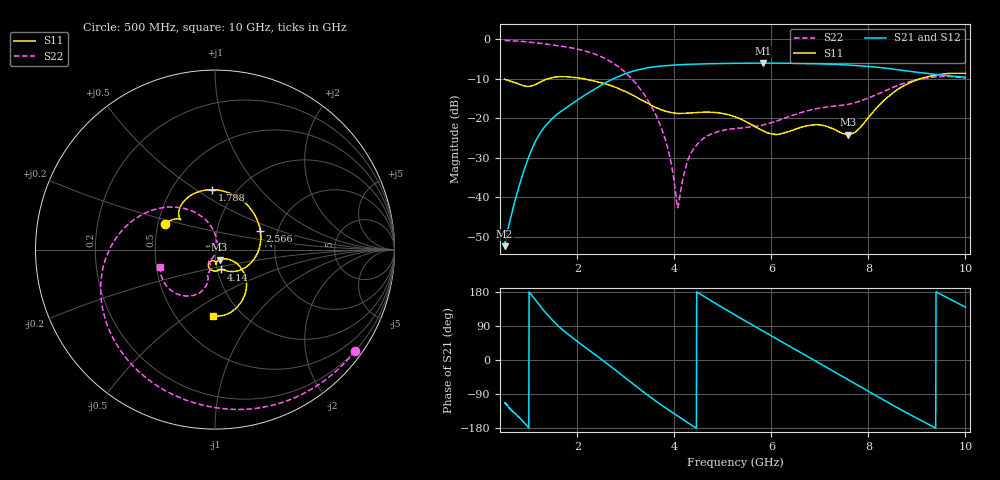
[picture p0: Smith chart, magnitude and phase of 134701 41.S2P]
!  2-Port S-parameters saved by WinCal
! VAR MeasName=S-Parameters (CALIBRATED_DATA) read from VNA (N5242A)
! VAR MeasDate=2013-7-3 16:37:49
! VAR NAME=134701 41
! VAR FILENAME=134701 41.S2P
! VAR DATE=2013-7-3 16:37:49
! VAR PHYS_PORTS=1,2
# Hz S MA R 50
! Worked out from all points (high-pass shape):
!   1601 points, 500 MHz to 10 GHz, reference 50 ohm
!   highest |S21| = -6.05 dB at 5.832 GHz (marker M1); lowest = -52.3 dB at 500 MHz (marker M2)
!   |S21| within 3 dB of the highest: 2.921 GHz to 9.508 GHz (6.587 GHz wide, 106 % of centre)
!   lowest |S11| = -24.2 dB at 7.589 GHz (marker M3), VSWR 1.13, Z = 52.3 - j5.93 ohm
!   |S11| at or under -10 dB: start of sweep to 1.39 GHz; 2.124 GHz to 9.07 GHz (6.946 GHz wide, 124 % of centre)
!   |S22| runs from -42.6 to -0.3 dB; largest |S21 - S12| = 0.0024
!   S11 on the Smith chart (normalised r, x): 500 MHz: 0.55, +0.18; 1.788 GHz: 0.78, +0.58; 2.566 GHz: 1.62, +0.37; 4.14 GHz: 1.04, -0.23; 10 GHz: 0.75, -0.64
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5e8  0.3117 152.4  0.002417 -112.9  0.002357 -110.7  0.9629 -35.9
7.909375e8  0.2708 140.6  0.01342 -151.1  0.01332 -150.9  0.9438 -56.5
1.09375e9  0.2606 138.7  0.04517 165.3  0.04504 165.1  0.9083 -77.9
1.360938e9  0.312 127.2  0.08274 122.3  0.08271 122.1  0.8653 -96.2
1.788438e9  0.3344 92.7  0.1386 69.8  0.1382 69.6  0.7924 -125.2
2.085312e9  0.3192 67.0  0.1838 40.6  0.1832 40.7  0.7284 -146.4
2.56625e9  0.2735 22.6  0.2779 -5.1  0.2778 -5.0  0.5717 176.6
3.035312e9  0.2112 -21.7  0.3744 -51.8  0.3745 -51.7  0.3569 138.5
3.670625e9  0.1327 -62.4  0.4538 -113.3  0.4534 -113.2  0.09357 91.2
3.890312e9  0.1196 -68.7  0.4658 -132.9  0.4664 -132.9  0.03596 71.7
4.056562e9  0.1154 -72.0  0.4727 -147.1  0.4731 -147.2  0.007987 7.4
4.139688e9  0.1152 -73.4  0.4761 -154.1  0.4761 -154.1  0.01298 -72.2
4.288125e9  0.1164 -77.2  0.4799 -166.4  0.4808 -166.4  0.03075 -95.5
4.495938e9  0.1184 -83.1  0.4845 176.9  0.4852 176.9  0.04893 -107.1
5.25e9  0.1045 -109.4  0.4953 119.0  0.4953 119.0  0.07422 -117.4
5.831875e9  0.06923 -111.0  0.4981 76.0  0.4982 75.9  0.08252 -109.8
6.372188e9  0.06844 -87.8  0.4955 36.5  0.4964 36.4  0.1058 -103.3
6.835312e9  0.08184 -85.3  0.4906 2.7  0.4903 2.7  0.1291 -104.9
7.589375e9  0.06188 -65.9  0.4696 -52.4  0.4707 -52.5  0.1505 -105.8
8.420625e9  0.19 -36.8  0.4252 -113.4  0.4247 -113.3  0.2332 -106.4
9.162812e9  0.3281 -63.9  0.3714 -164.6  0.372 -164.6  0.3214 -128.5
1e10  0.369 -91.5  0.3317 139.5  0.3323 139.6  0.3211 -162.1
